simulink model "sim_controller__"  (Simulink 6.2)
settings: Solver=ode3  StartTime=0.0  StopTime=70  RelTol=1e-3

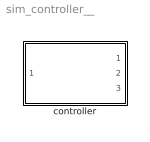
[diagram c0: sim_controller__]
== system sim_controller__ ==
  controller : Subsystem  Orientation=left

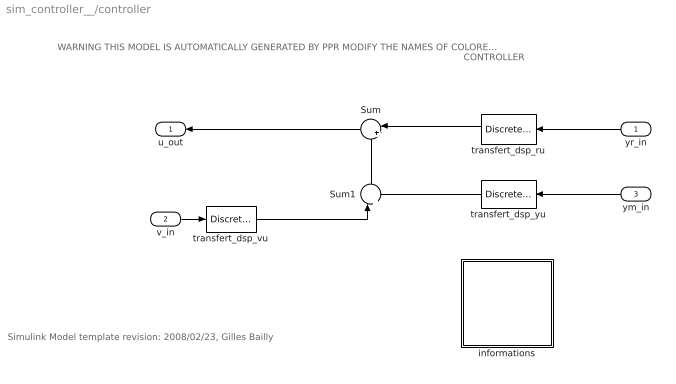
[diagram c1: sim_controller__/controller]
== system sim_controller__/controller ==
  note: Simulink Model template revision: 2008/02/23, Gilles Bailly
  note: CONTROLLER
  note: WARNING THIS MODEL IS AUTOMATICALLY GENERATED BY PPR MODIFY THE NAMES OF COLORED BLOCKS BREAK THIS LINK
  yr_in : Inport  Orientation=left  Port=1  LatchInput=off
  v_in : Inport  Port=2  LatchInput=off
  ym_in : Inport  Orientation=left  Port=3  LatchInput=off
  Sum : Sum  Orientation=left  Inputs=|+-
  Sum1 : Sum  Orientation=up  Inputs=|++
  informations : Subsystem
  transfert_dsp_ru : DiscreteFilter  Orientation=left  Numerator=[0 1.696627821]  Denominator=[1 -0.5384615385]  SampleTime=0.2
  transfert_dsp_vu : DiscreteFilter  Numerator=[0 0.4850813891 -1.390675476 1.348909365 -0.4437738546]  Denominator=[1 -3.597447204 4.883249106 -2.962402806 0.6770594807]  SampleTime=0.2
  transfert_dsp_yu : DiscreteFilter  Orientation=left  Numerator=[0 0.2359575101 -0.6549642993 0.6132367656 -0.1925442369]  Denominator=[1 -3.597447204 4.883249106 -2.962402806 0.6770594807]  SampleTime=0.2
  u_out : Outport  Orientation=left
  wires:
  transfert_dsp_vu/1 -> Sum1/1
  transfert_dsp_yu/1 -> Sum1/2
  Sum1/1 -> Sum/2
  yr_in/1 -> transfert_dsp_ru/1
  transfert_dsp_ru/1 -> Sum/1
  Sum/1 -> u_out/1
  ym_in/1 -> transfert_dsp_yu/1
  v_in/1 -> transfert_dsp_vu/1

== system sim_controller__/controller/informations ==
  note: info_annotation
